(* Logix 5000 AddOnInstructionDefinition export Banner_K50Audible_Param_v4; software revision 32.00; part 2 of 2 *)
(* tags used below, declared in another part *)
   K50 : Banner_K50Audible_v2;
   Port_Data : Banner_IOL_Port_v4;
   Port : DINT;
   Local_Control : DINT;
   Command_Being_Processed : BOOL;
   Update_Archive : BOOL;
   Index_Write_Inprocess : INT;
   Inprocess_Index : DINT;
   SP_Index : DINT;   // State Parameters Index
   SP_W_Index : DINT;
(* Banner_K50Audible_Param_v4, continued *)

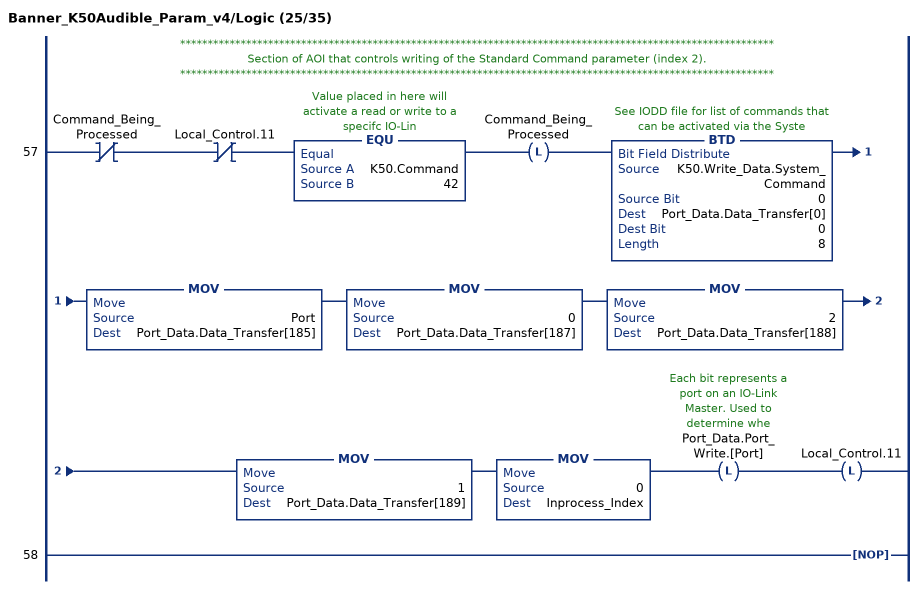
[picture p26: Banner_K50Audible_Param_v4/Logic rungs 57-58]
   // ************************************************************************************************************
   // Section of AOI that controls writing of the Standard Command parameter (index 2).
   // ************************************************************************************************************
   57: XIO(Command_Being_Processed)XIO(Local_Control.11)EQU(K50.Command,42)OTL(Command_Being_Processed)BTD(K50.Write_Data.System_Command,0,Port_Data.Data_Transfer[0],0,8)MOV(Port,Port_Data.Data_Transfer[185])MOV(0,Port_Data.Data_Transfer[187])MOV(2,Port_Data.Data_Transfer[188])MOV(1,Port_Data.Data_Transfer[189])MOV(0,Inprocess_Index)OTL(Port_Data.Port_Write.[Port])OTL(Local_Control.11);
   58: NOP();
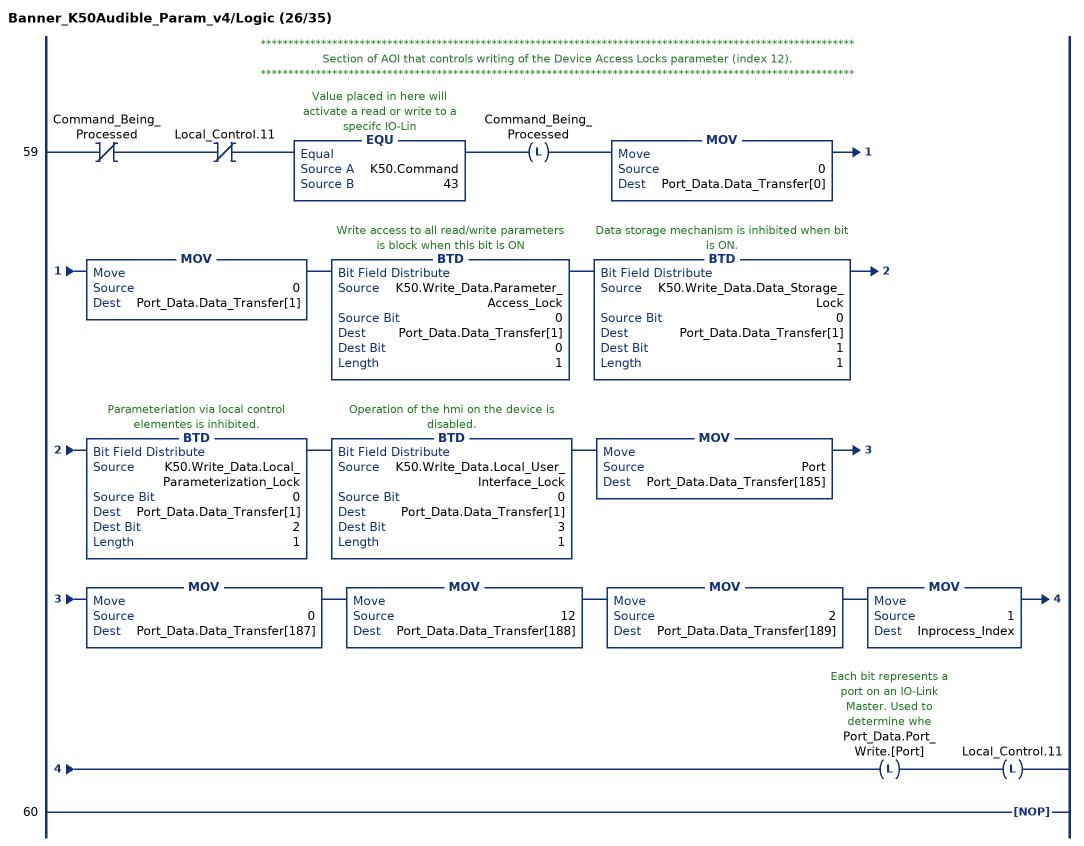
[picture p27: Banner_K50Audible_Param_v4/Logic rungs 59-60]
   // ************************************************************************************************************
   // Section of AOI that controls writing of the Device Access Locks parameter (index 12).
   // ************************************************************************************************************
   59: XIO(Command_Being_Processed)XIO(Local_Control.11)EQU(K50.Command,43)OTL(Command_Being_Processed)MOV(0,Port_Data.Data_Transfer[0])MOV(0,Port_Data.Data_Transfer[1])BTD(K50.Write_Data.Parameter_Access_Lock,0,Port_Data.Data_Transfer[1],0,1)BTD(K50.Write_Data.Data_Storage_Lock,0,Port_Data.Data_Transfer[1],1,1)BTD(K50.Write_Data.Local_Parameterization_Lock,0,Port_Data.Data_Transfer[1],2,1)BTD(K50.Write_Data.Local_User_Interface_Lock,0,Port_Data.Data_Transfer[1],3,1)MOV(Port,Port_Data.Data_Transfer[185])MOV(0,Port_Data.Data_Transfer[187])MOV(12,Port_Data.Data_Transfer[188])MOV(2,Port_Data.Data_Transfer[189])MOV(1,Inprocess_Index)OTL(Port_Data.Port_Write.[Port])OTL(Local_Control.11);
   60: NOP();
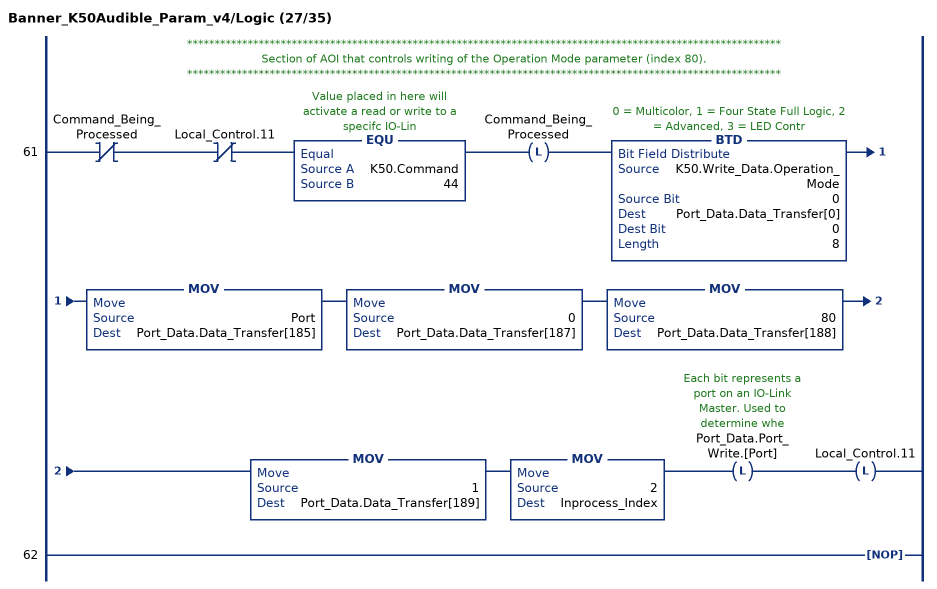
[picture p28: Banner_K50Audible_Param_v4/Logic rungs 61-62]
   // ************************************************************************************************************
   // Section of AOI that controls writing of the Operation Mode parameter (index 80).
   // ************************************************************************************************************
   61: XIO(Command_Being_Processed)XIO(Local_Control.11)EQU(K50.Command,44)OTL(Command_Being_Processed)BTD(K50.Write_Data.Operation_Mode,0,Port_Data.Data_Transfer[0],0,8)MOV(Port,Port_Data.Data_Transfer[185])MOV(0,Port_Data.Data_Transfer[187])MOV(80,Port_Data.Data_Transfer[188])MOV(1,Port_Data.Data_Transfer[189])MOV(2,Inprocess_Index)OTL(Port_Data.Port_Write.[Port])OTL(Local_Control.11);
   62: NOP();
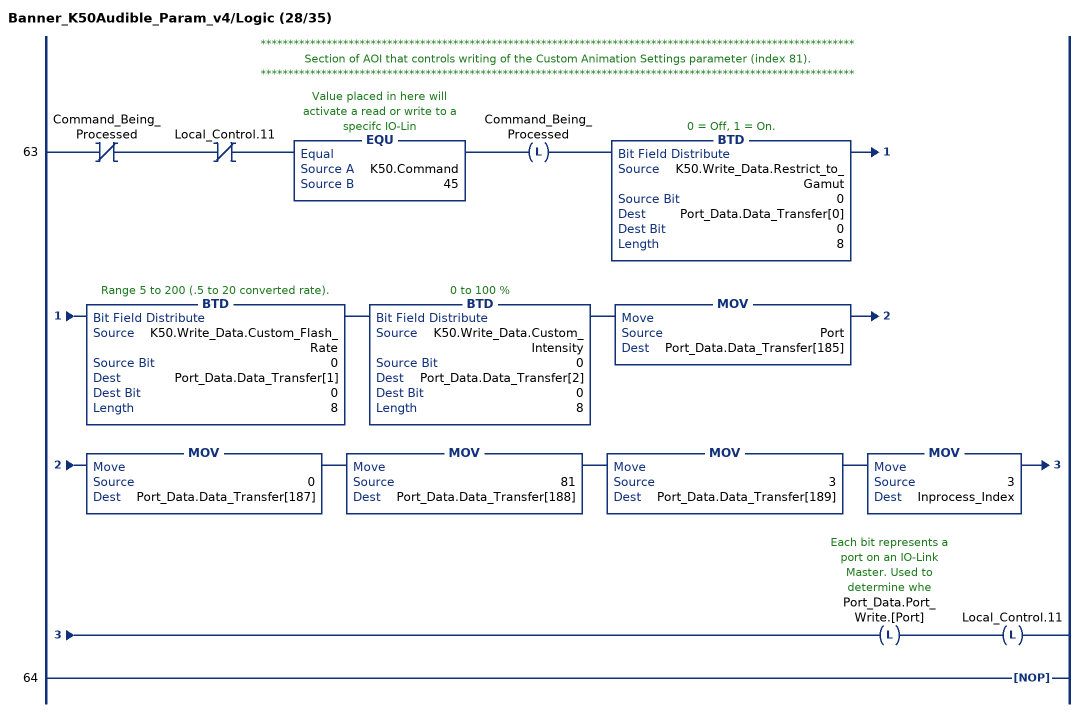
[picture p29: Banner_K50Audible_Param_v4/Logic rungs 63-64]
   // ************************************************************************************************************
   // Section of AOI that controls writing of the Custom Animation Settings parameter (index 81).
   // ************************************************************************************************************
   63: XIO(Command_Being_Processed)XIO(Local_Control.11)EQU(K50.Command,45)OTL(Command_Being_Processed)BTD(K50.Write_Data.Restrict_to_Gamut,0,Port_Data.Data_Transfer[0],0,8)BTD(K50.Write_Data.Custom_Flash_Rate,0,Port_Data.Data_Transfer[1],0,8)BTD(K50.Write_Data.Custom_Intensity,0,Port_Data.Data_Transfer[2],0,8)MOV(Port,Port_Data.Data_Transfer[185])MOV(0,Port_Data.Data_Transfer[187])MOV(81,Port_Data.Data_Transfer[188])MOV(3,Port_Data.Data_Transfer[189])MOV(3,Inprocess_Index)OTL(Port_Data.Port_Write.[Port])OTL(Local_Control.11);
   64: NOP();
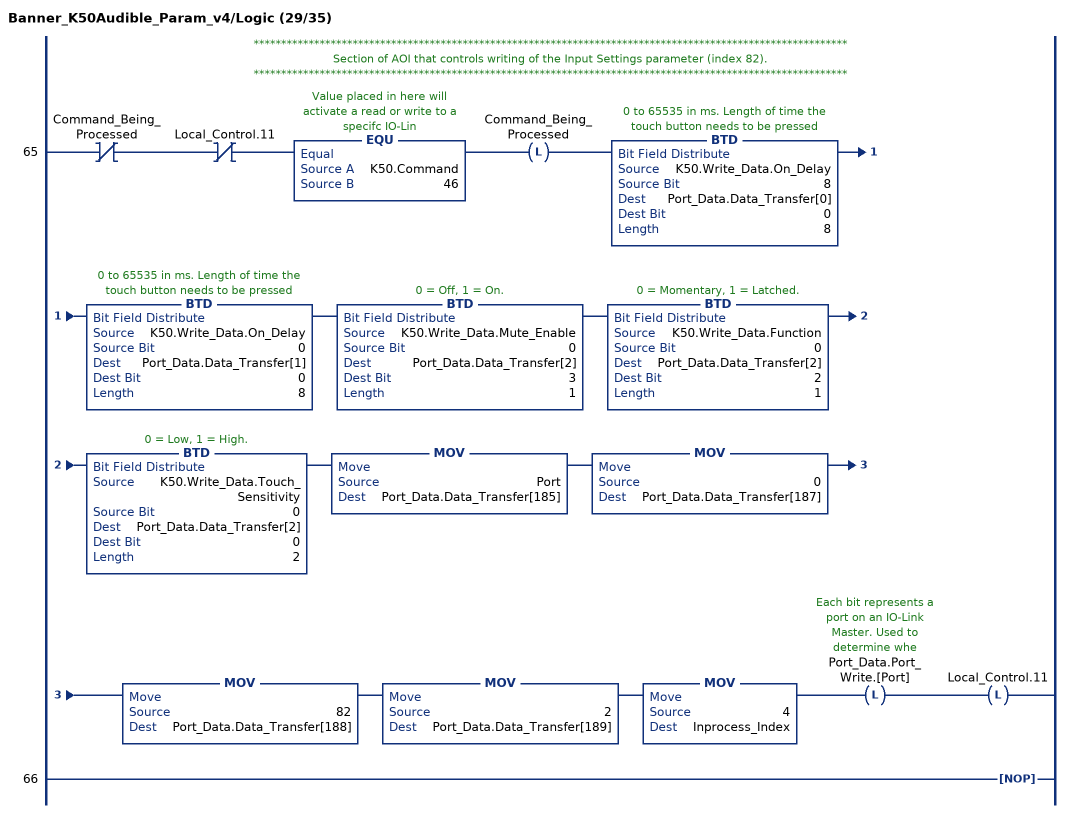
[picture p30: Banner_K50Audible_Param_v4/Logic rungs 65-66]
   // ************************************************************************************************************
   // Section of AOI that controls writing of the Input Settings parameter (index 82).
   // ************************************************************************************************************
   65: XIO(Command_Being_Processed)XIO(Local_Control.11)EQU(K50.Command,46)OTL(Command_Being_Processed)BTD(K50.Write_Data.On_Delay,8,Port_Data.Data_Transfer[0],0,8)BTD(K50.Write_Data.On_Delay,0,Port_Data.Data_Transfer[1],0,8)BTD(K50.Write_Data.Mute_Enable,0,Port_Data.Data_Transfer[2],3,1)BTD(K50.Write_Data.Function,0,Port_Data.Data_Transfer[2],2,1)BTD(K50.Write_Data.Touch_Sensitivity,0,Port_Data.Data_Transfer[2],0,2)MOV(Port,Port_Data.Data_Transfer[185])MOV(0,Port_Data.Data_Transfer[187])MOV(82,Port_Data.Data_Transfer[188])MOV(2,Port_Data.Data_Transfer[189])MOV(4,Inprocess_Index)OTL(Port_Data.Port_Write.[Port])OTL(Local_Control.11);
   66: NOP();
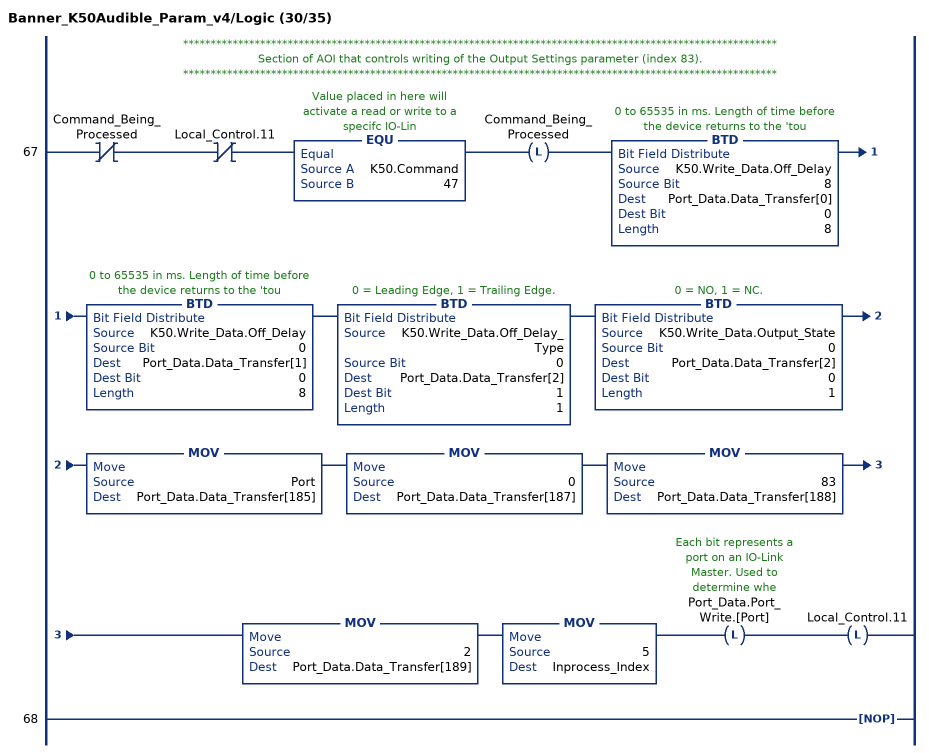
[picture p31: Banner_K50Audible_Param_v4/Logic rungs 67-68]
   // ************************************************************************************************************
   // Section of AOI that controls writing of the Output Settings parameter (index 83).
   // ************************************************************************************************************
   67: XIO(Command_Being_Processed)XIO(Local_Control.11)EQU(K50.Command,47)OTL(Command_Being_Processed)BTD(K50.Write_Data.Off_Delay,8,Port_Data.Data_Transfer[0],0,8)BTD(K50.Write_Data.Off_Delay,0,Port_Data.Data_Transfer[1],0,8)BTD(K50.Write_Data.Off_Delay_Type,0,Port_Data.Data_Transfer[2],1,1)BTD(K50.Write_Data.Output_State,0,Port_Data.Data_Transfer[2],0,1)MOV(Port,Port_Data.Data_Transfer[185])MOV(0,Port_Data.Data_Transfer[187])MOV(83,Port_Data.Data_Transfer[188])MOV(2,Port_Data.Data_Transfer[189])MOV(5,Inprocess_Index)OTL(Port_Data.Port_Write.[Port])OTL(Local_Control.11);
   68: NOP();
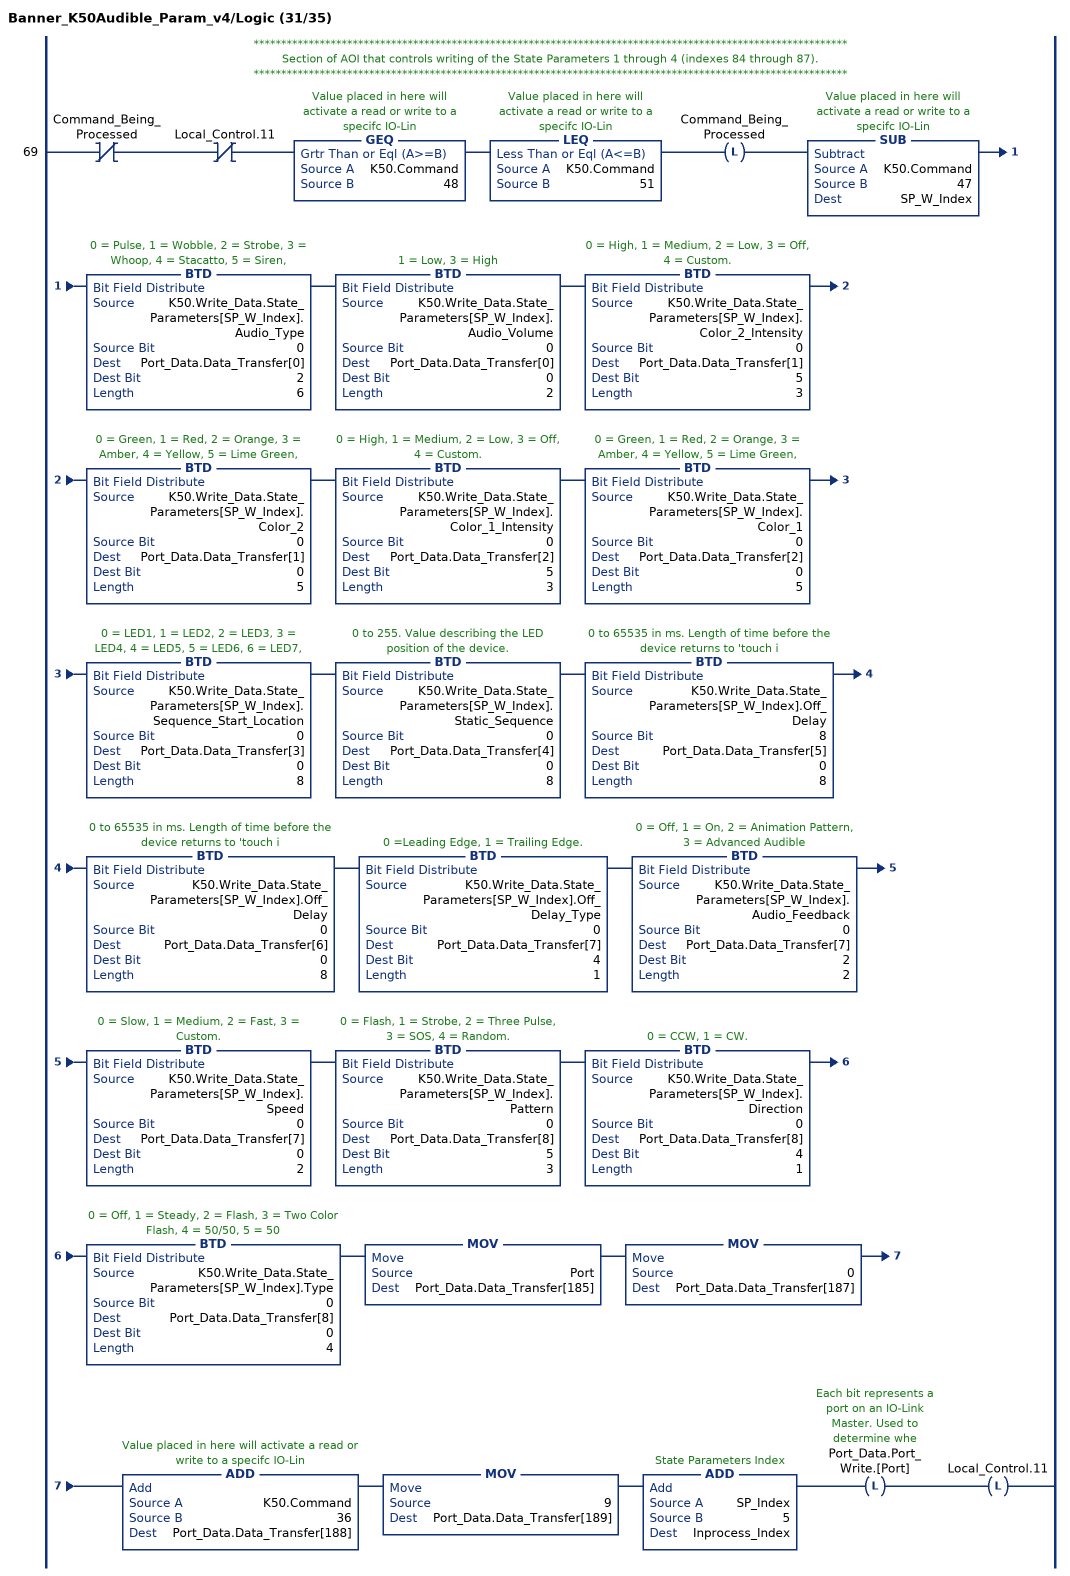
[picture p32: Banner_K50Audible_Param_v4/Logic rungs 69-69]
   // ************************************************************************************************************
   // Section of AOI that controls writing of the State Parameters 1 through 4 (indexes 84 through 87).
   // ************************************************************************************************************
   69: XIO(Command_Being_Processed)XIO(Local_Control.11)GEQ(K50.Command,48)LEQ(K50.Command,51)OTL(Command_Being_Processed)SUB(K50.Command,47,SP_W_Index)BTD(K50.Write_Data.State_Parameters[SP_W_Index].Audio_Type,0,Port_Data.Data_Transfer[0],2,6)BTD(K50.Write_Data.State_Parameters[SP_W_Index].Audio_Volume,0,Port_Data.Data_Transfer[0],0,2)BTD(K50.Write_Data.State_Parameters[SP_W_Index].Color_2_Intensity,0,Port_Data.Data_Transfer[1],5,3)BTD(K50.Write_Data.State_Parameters[SP_W_Index].Color_2,0,Port_Data.Data_Transfer[1],0,5)BTD(K50.Write_Data.State_Parameters[SP_W_Index].Color_1_Intensity,0,Port_Data.Data_Transfer[2],5,3)BTD(K50.Write_Data.State_Parameters[SP_W_Index].Color_1,0,Port_Data.Data_Transfer[2],0,5)BTD(K50.Write_Data.State_Parameters[SP_W_Index].Sequence_Start_Location,0,Port_Data.Data_Transfer[3],0,8)BTD(K50.Write_Data.State_Parameters[SP_W_Index].Static_Sequence,0,Port_Data.Data_Transfer[4],0,8)BTD(K50.Write_Data.State_Parameters[SP_W_Index].Off_Delay,8,Port_Data.Data_Transfer[5],0,8)BTD(K50.Write_Data.State_Parameters[SP_W_Index].Off_Delay,0,Port_Data.Data_Transfer[6],0,8)BTD(K50.Write_Data.State_Parameters[SP_W_Index].Off_Delay_Type,0,Port_Data.Data_Transfer[7],4,1)BTD(K50.Write_Data.State_Parameters[SP_W_Index].Audio_Feedback,0,Port_Data.Data_Transfer[7],2,2)BTD(K50.Write_Data.State_Parameters[SP_W_Index].Speed,0,Port_Data.Data_Transfer[7],0,2)BTD(K50.Write_Data.State_Parameters[SP_W_Index].Pattern,0,Port_Data.Data_Transfer[8],5,3)BTD(K50.Write_Data.State_Parameters[SP_W_Index].Direction,0,Port_Data.Data_Transfer[8],4,1)BTD(K50.Write_Data.State_Parameters[SP_W_Index].Type,0,Port_Data.Data_Transfer[8],0,4)MOV(Port,Port_Data.Data_Transfer[185])MOV(0,Port_Data.Data_Transfer[187])ADD(K50.Command,36,Port_Data.Data_Transfer[188])MOV(9,Port_Data.Data_Transfer[189])ADD(SP_Index,5,Inprocess_Index)OTL(Port_Data.Port_Write.[Port])OTL(Local_Control.11);
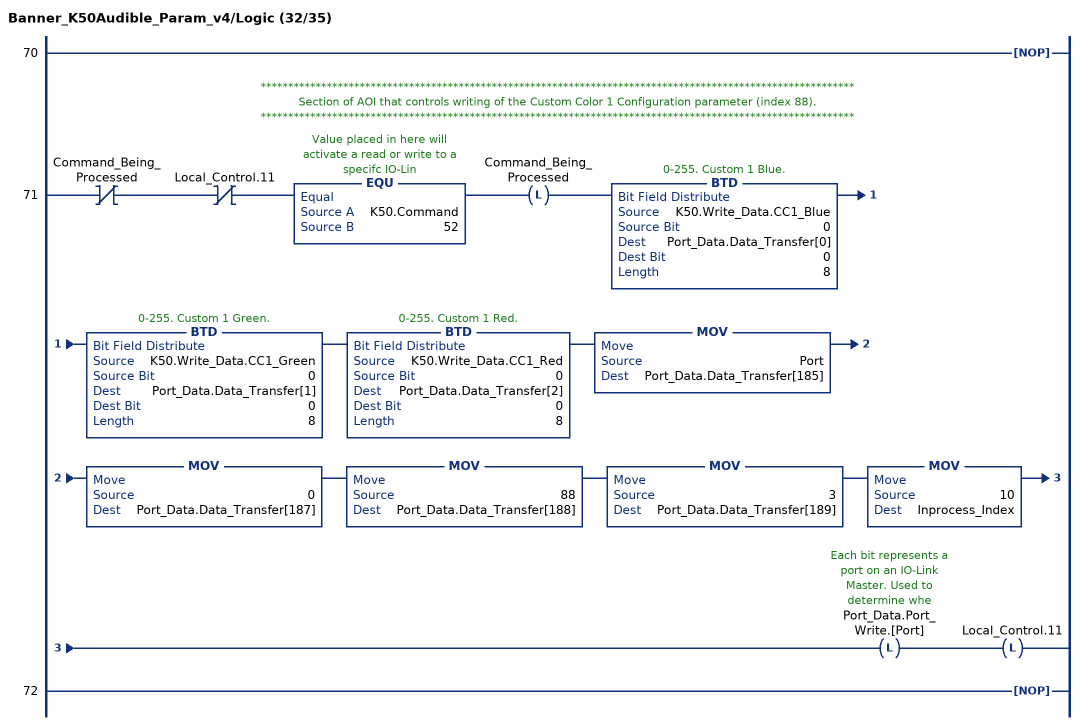
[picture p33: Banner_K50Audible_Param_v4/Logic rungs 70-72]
   70: NOP();
   // ************************************************************************************************************
   // Section of AOI that controls writing of the Custom Color 1 Configuration parameter (index 88).
   // ************************************************************************************************************
   71: XIO(Command_Being_Processed)XIO(Local_Control.11)EQU(K50.Command,52)OTL(Command_Being_Processed)BTD(K50.Write_Data.CC1_Blue,0,Port_Data.Data_Transfer[0],0,8)BTD(K50.Write_Data.CC1_Green,0,Port_Data.Data_Transfer[1],0,8)BTD(K50.Write_Data.CC1_Red,0,Port_Data.Data_Transfer[2],0,8)MOV(Port,Port_Data.Data_Transfer[185])MOV(0,Port_Data.Data_Transfer[187])MOV(88,Port_Data.Data_Transfer[188])MOV(3,Port_Data.Data_Transfer[189])MOV(10,Inprocess_Index)OTL(Port_Data.Port_Write.[Port])OTL(Local_Control.11);
   72: NOP();
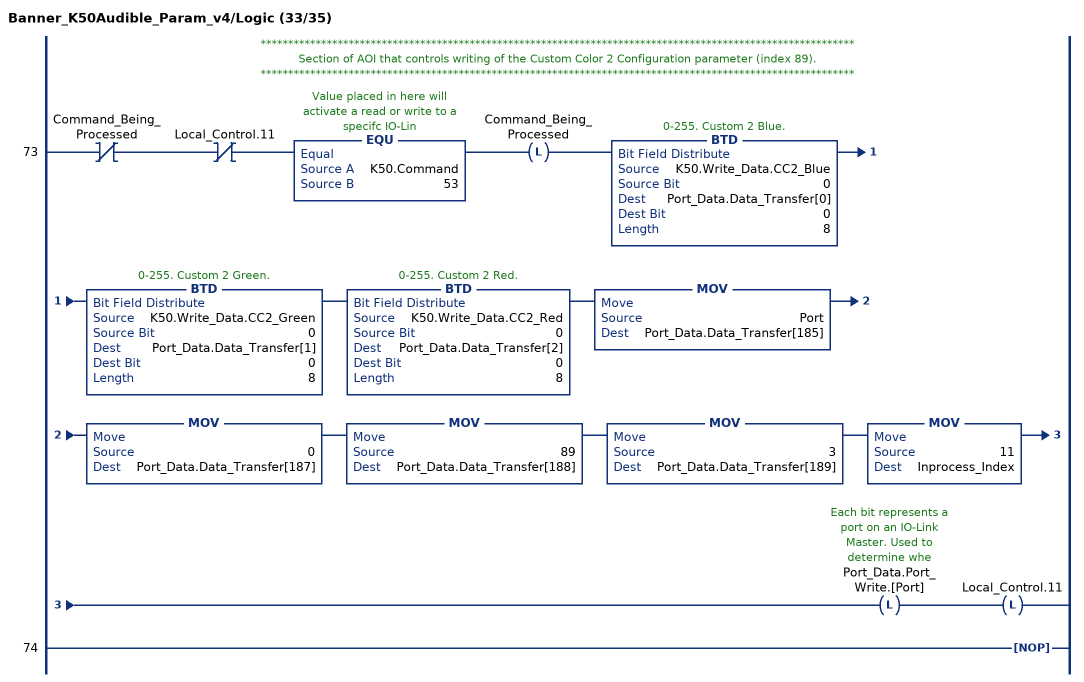
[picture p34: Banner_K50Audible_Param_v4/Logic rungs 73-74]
   // ************************************************************************************************************
   // Section of AOI that controls writing of the Custom Color 2 Configuration parameter (index 89).
   // ************************************************************************************************************
   73: XIO(Command_Being_Processed)XIO(Local_Control.11)EQU(K50.Command,53)OTL(Command_Being_Processed)BTD(K50.Write_Data.CC2_Blue,0,Port_Data.Data_Transfer[0],0,8)BTD(K50.Write_Data.CC2_Green,0,Port_Data.Data_Transfer[1],0,8)BTD(K50.Write_Data.CC2_Red,0,Port_Data.Data_Transfer[2],0,8)MOV(Port,Port_Data.Data_Transfer[185])MOV(0,Port_Data.Data_Transfer[187])MOV(89,Port_Data.Data_Transfer[188])MOV(3,Port_Data.Data_Transfer[189])MOV(11,Inprocess_Index)OTL(Port_Data.Port_Write.[Port])OTL(Local_Control.11);
   74: NOP();
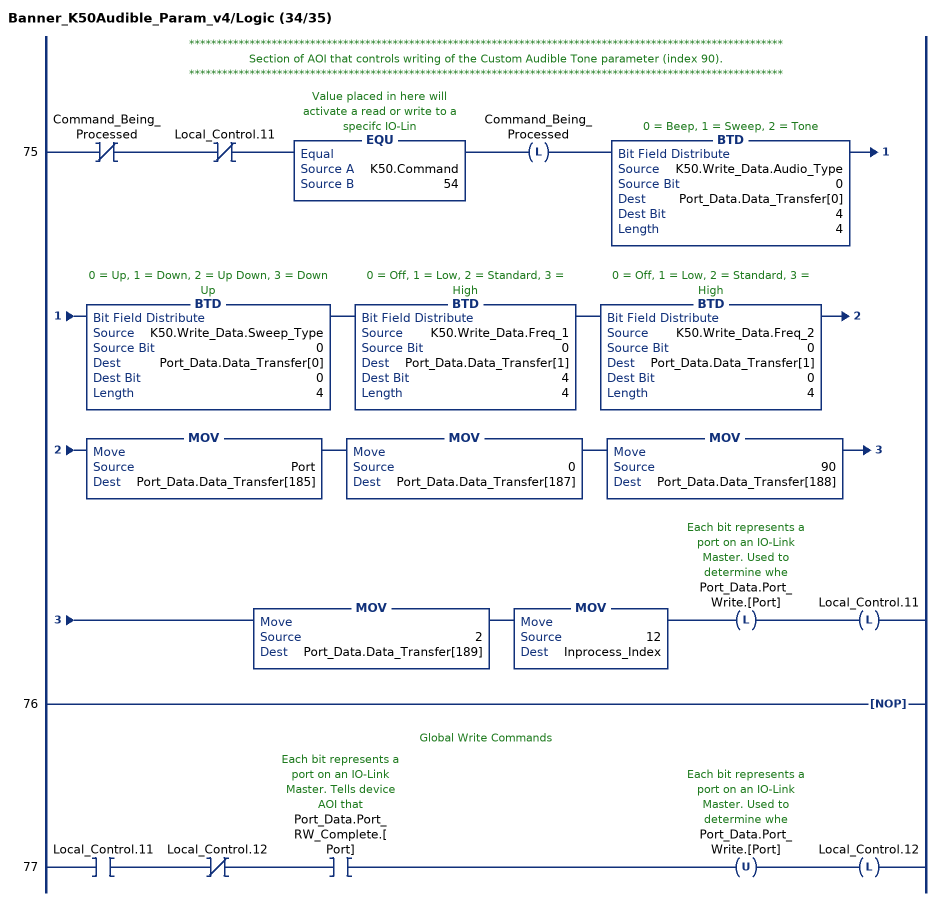
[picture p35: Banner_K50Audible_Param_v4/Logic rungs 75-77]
   // ************************************************************************************************************
   // Section of AOI that controls writing of the Custom Audible Tone parameter (index 90).
   // ************************************************************************************************************
   75: XIO(Command_Being_Processed)XIO(Local_Control.11)EQU(K50.Command,54)OTL(Command_Being_Processed)BTD(K50.Write_Data.Audio_Type,0,Port_Data.Data_Transfer[0],4,4)BTD(K50.Write_Data.Sweep_Type,0,Port_Data.Data_Transfer[0],0,4)BTD(K50.Write_Data.Freq_1,0,Port_Data.Data_Transfer[1],4,4)BTD(K50.Write_Data.Freq_2,0,Port_Data.Data_Transfer[1],0,4)MOV(Port,Port_Data.Data_Transfer[185])MOV(0,Port_Data.Data_Transfer[187])MOV(90,Port_Data.Data_Transfer[188])MOV(2,Port_Data.Data_Transfer[189])MOV(12,Inprocess_Index)OTL(Port_Data.Port_Write.[Port])OTL(Local_Control.11);
   76: NOP();
   // Global Write Commands
   77: XIC(Local_Control.11)XIO(Local_Control.12)XIC(Port_Data.Port_RW_Complete.[Port])OTU(Port_Data.Port_Write.[Port])OTL(Local_Control.12);
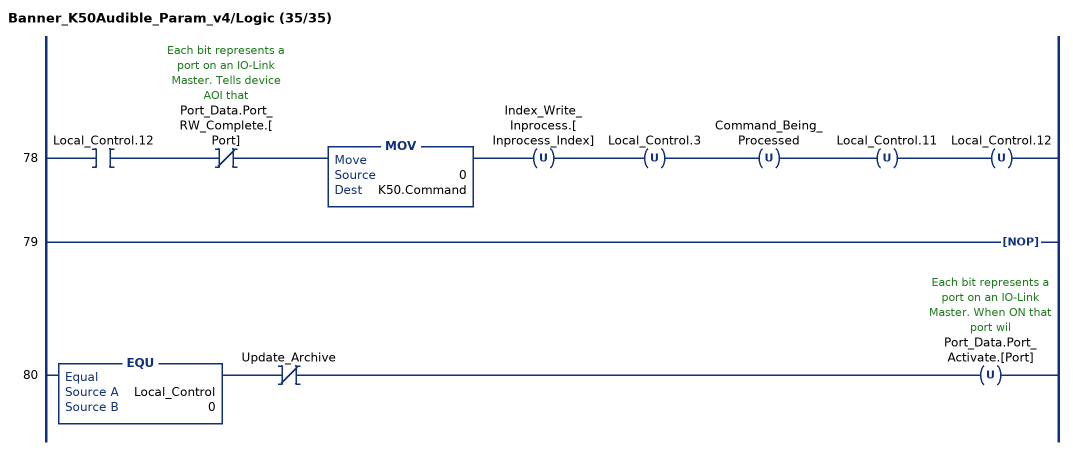
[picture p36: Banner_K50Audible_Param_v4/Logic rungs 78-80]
   78: XIC(Local_Control.12)XIO(Port_Data.Port_RW_Complete.[Port])MOV(0,K50.Command)OTU(Index_Write_Inprocess.[Inprocess_Index])OTU(Local_Control.3)OTU(Command_Being_Processed)OTU(Local_Control.11)OTU(Local_Control.12);
   79: NOP();
   80: EQU(Local_Control,0)XIO(Update_Archive)OTU(Port_Data.Port_Activate.[Port]);
END_ROUTINE
END_ADD_ON_INSTRUCTION
